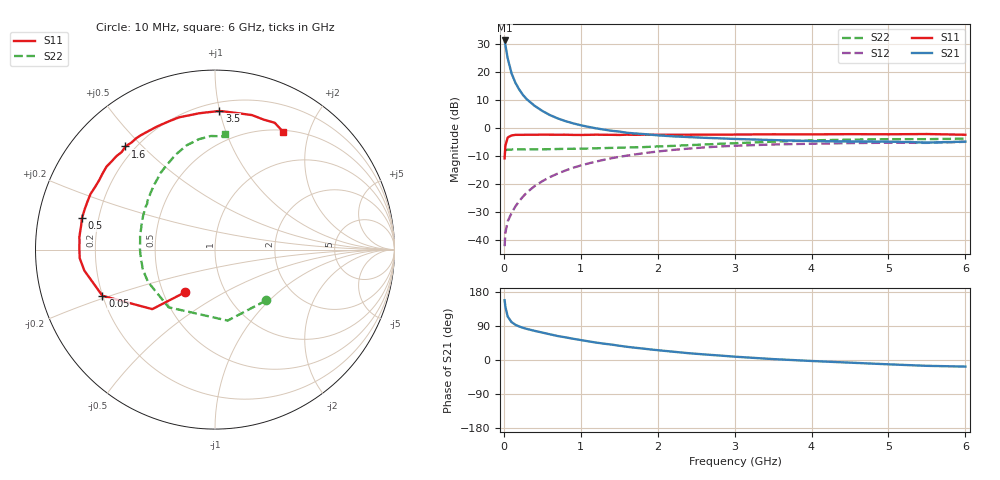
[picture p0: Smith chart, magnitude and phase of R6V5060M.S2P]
! SIEMENS Small Signal Semiconductors
! BFR193
! Si NPN RF Bipolar Junction Transistor in SOT23
! VCE = 0.5 V  IC = 60 mA
! Common Emitter S-Parameters:  May  1996
# GHz  S  MA  R  50
!  f  S11  S21  S12  S22
! GHz  MAG  ANG  MAG  ANG  MAG  ANG  MAG  ANG
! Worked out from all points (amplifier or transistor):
!   36 points, 10 MHz to 6 GHz, reference 50 ohm
!   highest |S21| = 31.2 dB at 10 MHz (marker M1)
!   |S21| within 3 dB of that: start of sweep to 29.06 MHz
!   unconditionally stable (mu >= 1): start of sweep to 16.95 MHz; 121.5 MHz to end of sweep
!   at 250 MHz: K = 1.15, MAG = 15.7 dB, |S12| = -24.4 dB
!   at 1.4 GHz: K = 1.11, MAG = 2.9 dB, |S12| = -10.8 dB
!   at 6 GHz: K = 1.03, MAG = -1.1 dB, |S12| = -4.9 dB
!   S11 on the Smith chart (normalised r, x): 10 MHz: 0.65, -0.34; 50 MHz: 0.20, -0.19; 500 MHz: 0.14, +0.12; 1.6 GHz: 0.16, +0.45; 3.5 GHz: 0.26, +1.00; 6 GHz: 0.52, +1.61
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0.01  0.2891 -124.9  36.12 157.7  0.0079 63.6  0.4017 -44.9
0.02  0.4818 -136.5  30.19 140.5  0.0137 57.7  0.4018 -79.9
0.05  0.678 -157.7  17.42 114.7  0.0218 51.7  0.4124 -128.8
0.1  0.7374 -170.9  9.406 100.0  0.0307 56.4  0.4145 -154.3
0.15  0.7554 -176.4  6.387 93.0  0.0402 62.2  0.4173 -164.4
0.2  0.7558 179.4  4.839 88.4  0.0502 65.4  0.4148 -169.8
0.25  0.7562 176.9  3.857 84.8  0.0604 67.2  0.416 -173.8
0.3  0.7589 174.5  3.233 82.0  0.0716 68.6  0.4165 -176.4
0.4  0.7577 169.8  2.481 76.9  0.0925 69.0  0.4183 179.4
0.5  0.7618 166.6  2.016 72.4  0.1132 68.6  0.4185 175.9
0.6  0.76 162.6  1.696 67.8  0.1341 67.5  0.4201 173.0
0.7  0.7593 159.0  1.483 63.3  0.1546 66.0  0.4231 170.5
0.9  0.7536 152.4  1.211 56.1  0.1961 62.6  0.4268 165.4
1.1  0.7561 146.1  1.047 49.2  0.2345 58.8  0.4325 161.2
1.3  0.7571 139.5  0.937 43.1  0.2719 54.7  0.4392 156.5
1.6  0.7612 131.0  0.823 34.9  0.3224 48.5  0.4516 150.3
2.2  0.7582 115.1  0.711 21.9  0.4079 36.3  0.4808 137.7
2.6  0.7636 105.2  0.67 14.8  0.4509 28.5  0.5073 129.3
3.5  0.7729 88.2  0.61 2.4  0.5094 12.9  0.5716 112.8
4.5  0.7772 74.6  0.576 -7.0  0.5384 -0.2  0.6215 98.3
5.5  0.7811 64.8  0.551 -15.4  0.5437 -11.5  0.6333 84.6
6  0.7586 60.1  0.572 -17.4  0.5673 -15.1  0.6473 85.0
